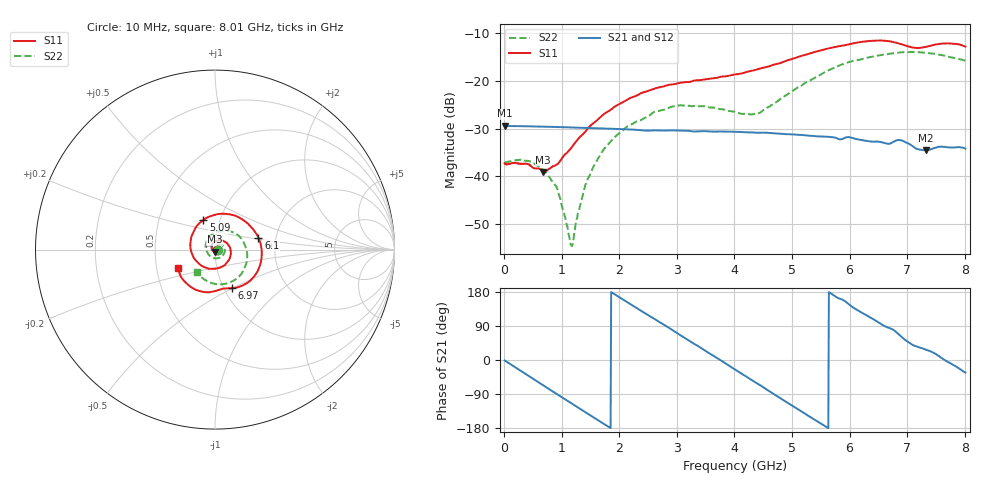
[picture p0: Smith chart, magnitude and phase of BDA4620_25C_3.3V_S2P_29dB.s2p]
!Agilent Technologies,E5071B,MY42404982,A.09.10
!Date: Wed May 06 08:55:08 2026
!Data & Calibration Information:
!Freq	S11:SOLT2(ON)	S21:SOLT2(ON)	S12:SOLT2(ON)	S22:SOLT2(ON)
# Hz S RI R 50
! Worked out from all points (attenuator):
!   801 points, 10 MHz to 8.01 GHz, reference 50 ohm
!   highest |S21| = -29.37 dB at 10 MHz (marker M1); lowest = -34.5 dB at 7.32 GHz (marker M2)
!   lowest |S11| = -39.0 dB at 680 MHz (marker M3), VSWR 1.02, Z = 49.9 - j1.11 ohm
!   |S11| at or under -10 dB: start of sweep to end of sweep
!   |S22| runs from -54.6 to -13.9 dB; largest |S21 - S12| = 0.00017
!   S11 on the Smith chart (normalised r, x): 10 MHz: 1.03, -0.00; 5.09 GHz: 0.83, +0.28; 6.1 GHz: 1.62, +0.23; 6.97 GHz: 1.09, -0.50; 8.01 GHz: 0.65, -0.14
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1e7  0.0137 -0.000847  0.034 -0.000733  0.0341 -0.000698  0.014 -0.000505
4.2e8  0.00858 -0.0103  0.0252 -0.0222  0.0252 -0.0222  0.0136 -0.00495
6.8e8  -0.00109 -0.0111  0.0132 -0.0306  0.0131 -0.0306  0.00939 -0.00695
9.3e8  -0.0122 -0.00564  -0.000643 -0.0329  -0.000701 -0.033  0.00354 -0.00629
1.16e9  -0.0186 0.0065  -0.013 -0.0299  -0.013 -0.03  -0.00148 -0.00121
1.2e9  -0.0191 0.00907  -0.015 -0.0289  -0.015 -0.029  -0.00206 -3.19e-05
1.35e9  -0.0191 0.0192  -0.0216 -0.0241  -0.0216 -0.0241  -0.00362 0.00451
1.53e9  -0.014 0.0323  -0.0275 -0.0165  -0.0276 -0.0165  -0.00342 0.0112
1.77e9  0.00117 0.0464  -0.0314 -0.0044  -0.0315 -0.00438  0.000629 0.0205
2.15e9  0.0395 0.0509  -0.0274 0.0149  -0.0274 0.015  0.0169 0.0292
2.68e9  0.0853 0.00621  -0.00623 0.0297  -0.00622 0.0297  0.0442 0.0197
3.08e9  0.0798 -0.054  0.0133 0.0271  0.0135 0.0271  0.0551 -0.00708
4.01e9  -0.0772 -0.0883  0.0266 -0.0124  0.0267 -0.0124  -0.0102 -0.0465
4.42e9  -0.1337 -0.00581  0.0125 -0.0258  0.0125 -0.0259  -0.0441 -0.0128
5.09e9  -0.0651 0.1652  -0.0172 -0.0213  -0.0172 -0.0214  -0.0198 0.0826
5.35e9  0.0147 0.1976  -0.0238 -0.0118  -0.0238 -0.0119  0.0229 0.1017
6.1e9  0.2418 0.0665  -0.0175 0.0176  -0.0175 0.0176  0.1592 0.0419
6.68e9  0.1972 -0.172  0.00194 0.0219  0.002 0.0219  0.17 -0.0901
6.97e9  0.0962 -0.215  0.0139 0.0182  0.0139 0.0182  0.1304 -0.1528
7.32e9  0.0133 -0.2275  0.0166 0.00872  0.0167 0.00873  0.0481 -0.1921
7.65e9  -0.1078 -0.2234  0.0204 -8.72e-06  0.0204 -1.95e-05  -0.0328 -0.1811
8.01e9  -0.2051 -0.1042  0.0163 -0.0107  0.0164 -0.0108  -0.1016 -0.1275
